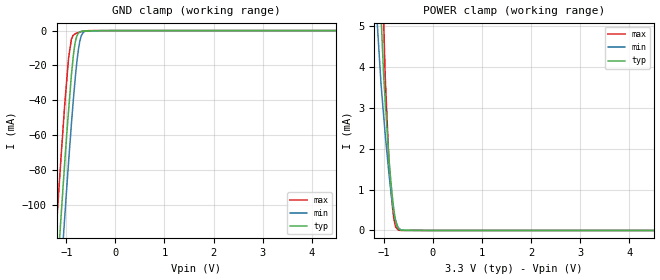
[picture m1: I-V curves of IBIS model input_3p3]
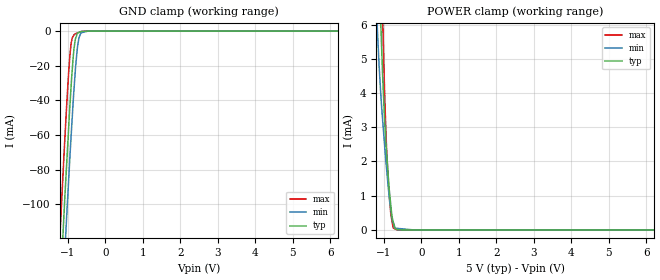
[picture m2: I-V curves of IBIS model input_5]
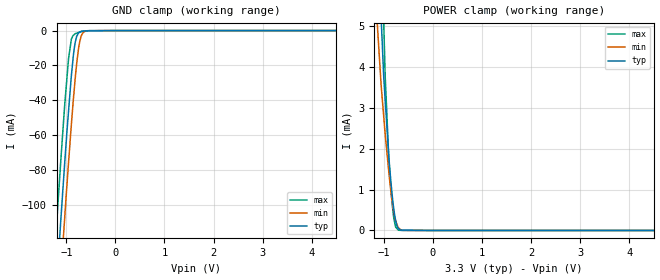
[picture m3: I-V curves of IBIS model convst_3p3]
|Texas Instruments Incorporated
| 18 Bit 1MSPS Parallel ADC W/Ref, Pseudo Bipolar, Fully Differential Input
| Marketing part#   Digital Voltage Range   Package-type   #pins
| ADS8482IBRGZR   2.7 - 5.25V   VQFN   48
| ADS8482IBRGZRG4   2.7 - 5.25V   VQFN   48
| ADS8482IBRGZT   2.7 - 5.25V   VQFN   48
| ADS8482IBRGZTG4   2.7 - 5.25V   VQFN   48
| ADS8482IRGZR   2.7 - 5.25V   VQFN   48
| ADS8482IRGZRG4   2.7 - 5.25V   VQFN   48
| ADS8482IRGZT   2.7 - 5.25V   VQFN   48
| ADS8482IRGZTG4   2.7 - 5.25V   VQFN   48
[IBIS Ver]   3.2
[File name]   ads8482.ibs
|SIMDE Ver   V2.2 - 201009 - RHL4 - Build 424
[File Rev]   1.1
[Date]   03/11/2011
[Source]
| Texas Instruments Incorporated.
| Analog-eLab Design Center, HPA
| 12500 TI Blvd
| Dallas, TX -75243
| e-mail: elab_ibis@list.ti.com
| -Model generated from simulations in TISPICE
[Notes]   Revision History:
| Rev 1.0: 1/21/2011
| - Initial version of the model
| - Model generated from simulations in TISPICE
| - Model matched to SPICE simulation
| - C_comp although listed in numerical order of value are
|   obtained from varying PVT conditions. For PVT conditions for
|   each specific value refer the buffer description under
|   respective [Model]. IBIS model user is responsible for using
|   appropriate C_comp to simulate for Signal Integrity.
| - Model names with a trailing _3p3 contains
|   the model for 3.3V [3.0V and 3.6V]. Model names with trailing _5
|   contains the model for 5.0V [4.75V and 5.25V] operation.
| Rev 1.1: 03/11/2011
| - Updated copyright to 2011
[Disclaimer]
| This model is designed as an aid for customers of Texas Instruments.
| TI and its licensors and suppliers make no warranties, either expressed
| or implied, with respect to this  model, including the warranties of
| merchantability or fitness for a particular purpose. The model is
| provided solely on an "as is" basis. The entire risk as to its quality
| and performance is with the customer.
[Copyright]
 (C) Copyright 2011 Texas Instruments Incorporated.All rights reserved.
|   ADS8482
[Component]   ADS8482
[Manufacturer]   TI
[Package]   |48 VQFN -  RGZ package
|   typ   min   max
R_pkg   0.08052   0.03771   0.10186
L_pkg   1.45674nH   0.98129nH   1.85620nH
C_pkg   0.15530pF   0.13533pF   0.18669pF
[Pin]  signal_name   model_name   R_pin   L_pin   C_pin
1   VBD   POWER   0.09317   1.68150nH  0.14766pF
2   BUS18/_16   input   0.08577   1.52984nH  0.15866pF
3   BYTE   input   0.07932   1.40125nH  0.15118pF
4   _CONVST   convst   0.03771   0.98129nH  0.18224pF
5   _RD   input   0.07064   1.23015nH  0.14114pF
6   _CS   input   0.06907   1.19953nH  0.13533pF
7   VA   POWER   0.06918   1.20163nH  0.13515pF
8   AGND   GND   0.06936   1.20524nH  0.13665pF
9   AGND   GND   0.07148   1.24671nH  0.13959pF
10   VA   POWER   0.07551   1.32594nH  0.14513pF
11   REFM   GND   0.08138   1.44284nH  0.15299pF
12   REFM   GND   0.08851   1.58840nH  0.14292pF
13   REFIN   TERM   0.04791   1.34371nH  0.18669pF
14   REFOUT   TERM   0.09373   1.68884nH  0.16643pF
15   NC   NC   0.08818   1.57624nH  0.15943pF
16   VA   POWER   0.08376   1.48731nH  0.15367pF
17   AGND   GND   0.08064   1.42465nH  0.14967pF
18   IN(+)   TERM   0.07903   1.39192nH  0.14762pF
19   IN(-)   TERM   0.07908   1.39202nH  0.14763pF
20   AGND   GND   0.08076   1.42454nH  0.14974pF
21   VA   POWER   0.08394   1.48721nH  0.15381pF
22   VA   POWER   0.08845   1.57664nH  0.15955pF
23   AGND   GND   0.09404   1.68894nH  0.16459pF
24   AGND   GND   0.09491   1.71030nH  0.14731pF
25   VA   POWER   0.04541   1.19009nH  0.19066pF
26   AGND   GND   0.08580   1.52394nH  0.16244pF
27   AGND   GND   0.04036   1.03065nH  0.19517pF
28   DB17   db   0.07628   1.33321nH  0.14727pF
29   DB16   db   0.07240   1.25624nH  0.14061pF
30   DB15   db   0.07047   1.21832nH  0.13804pF
31   DB14   db   0.07072   1.22312nH  0.13834pF
32   DB13   db   0.07310   1.27024nH  0.14147pF
33   DB12   db   0.07738   1.35501nH  0.14714pF
34   DB11   db   0.08319   1.47074nH  0.15496pF
35   DB10   db   0.09018   1.61144nH  0.16452pF
36   VBD   POWER   0.04686   1.31549nH  0.18631pF
37   BDGND   GND   0.04818   1.32883nH  0.18833pF
38   DB9   db   0.10081   1.82484nH  0.17209pF
39   DB8   db   0.09486   1.70495nH  0.16715pF
40   DB7   db   0.08995   1.60681nH  0.16090pF
41   DB6   db   0.08626   1.53385nH  0.15618pF
42   DB5   db   0.08401   1.48973nH  0.15334pF
43   DB4   db   0.08333   1.47703nH  0.15250pF
44   DB3   db   0.08427   1.49644nH  0.15371pF
45   DB2   db   0.08677   1.54701nH  0.15692pF
46   DB1   db   0.09066   1.62564nH  0.16196pF
47   DB0   db   0.09576   1.72934nH  0.16839pF
48   BUSY   busy   0.10186   1.85620nH  0.15594pF
[Pin Mapping]  pulldown_ref pullup_ref gnd_clamp_ref power_clamp_ref
1   NC   PWRBUS1
2   GNDBUS1   PWRBUS1
3   GNDBUS1   PWRBUS1
4   GNDBUS1   PWRBUS1
5   GNDBUS1   PWRBUS1
6   GNDBUS1   PWRBUS1
7   NC   PWRBUS2
8   GNDBUS2   NC
9   GNDBUS2   NC
10   NC   PWRBUS2
11   GNDBUS3   NC
12   GNDBUS3   NC
13   GNDBUS2   PWRBUS2
14   GNDBUS2   PWRBUS2
15   NC   NC
16   NC   PWRBUS2
17   GNDBUS2   NC
18   GNDBUS2   PWRBUS2
19   GNDBUS2   PWRBUS2
20   GNDBUS2   NC
21   NC   PWRBUS2
22   NC   PWRBUS2
23   GNDBUS2   NC
24   GNDBUS2   NC
25   NC   PWRBUS2
26   GNDBUS2   NC
27   GNDBUS2   NC
28   GNDBUS1   PWRBUS1
29   GNDBUS1   PWRBUS1
30   GNDBUS1   PWRBUS1
31   GNDBUS1   PWRBUS1
32   GNDBUS1   PWRBUS1
33   GNDBUS1   PWRBUS1
34   GNDBUS1   PWRBUS1
35   GNDBUS1   PWRBUS1
36   NC   PWRBUS1
37   GNDBUS1   NC
38   GNDBUS1   PWRBUS1
39   GNDBUS1   PWRBUS1
40   GNDBUS1   PWRBUS1
41   GNDBUS1   PWRBUS1
42   GNDBUS1   PWRBUS1
43   GNDBUS1   PWRBUS1
44   GNDBUS1   PWRBUS1
45   GNDBUS1   PWRBUS1
46   GNDBUS1   PWRBUS1
47   GNDBUS1   PWRBUS1
48   GNDBUS1   PWRBUS1
|   Model Selectors
[Model Selector] input
input_3p3   3.3V digital input
input_5   5.0V digital input
[Model Selector] convst
convst_3p3   3.3V digital input
convst_5   5.0V digital input
[Model Selector] busy
busy_3p3   3.3V digital output
busy_5   5.0V digital output
[Model Selector] db
db_3p3   3.3V 3-state output
db_5   5.0V 3-state output
[Model Selector] TERM
TERM_3p3  3.3V nominal termination
TERM_5   5.0V nominal termination
[Model]  TERM_3p3
Model_type Terminator
C_comp   1.0e-20F  1.0e-20F  1.0e-20F
|   typ   min   max
[Voltage Range]   3.3V   3.0V   3.6V
[POWER Clamp Reference]   3.3V   3.0V   3.6V
[GND Clamp Reference]   0V   0V   0V
|Ambient Temperature   25   85   -40
|Junction Temperature
[Temperature Range]   30   90   -40
[Model]  TERM_5
Model_type Terminator
C_comp   1.0e-20F  1.0e-20F  1.0e-20F
|   typ   min   max
[Voltage Range]   5.0V   4.75V   5.25V
[POWER Clamp Reference]   5.0V   4.75V   5.25V
[GND Clamp Reference]   0V   0V   0V
|Ambient Temperature   25   85   -40
|Junction Temperature
[Temperature Range]   30   90   -40
| Models and submodels in the file (10): input_3p3 (Input), input_5 (Input), convst_3p3 (Input), convst_5 (Input), busy_3p3 (Output), busy_5 (Output), db_3p3 (3-state), db_5 (3-state), TERM_3p3 (Terminator), TERM_5 (Terminator)
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|   input_3p3 Model
[Model]   input_3p3
Model_type   Input
Vinl = 0.8
Vinh = 2.3
|   typ   min   max
|   (nom PVT)   (Fast PVT)   (slow PVT)
|C_comp from frequency method(F=1MHz)
|Average
|C_comp   1.211e-12   1.085e-12   1.349e-12
|C_comp from L-C Tank method(L=1nH)
|Resonant Frequency(Hz)   5.36e9   5.44e9   5.26e9
C_comp   8.826e-13   8.568e-13   9.164e-13
| Where nom  PVT is Nominal Process,  3.3V,  30C
|   Fast PVT is Strong Process,   3.6V,  -40C
|   Slow PVT is Weak Process,   3V,  90C
[Model Spec]
Vinl   0.8   0.8   0.8
Vinh   2.3   2.0   2.6
[Voltage Range]   3.3   3   3.6
|Ambient Temperature   25   85   -40
|Junction Temperature
[Temperature Range]   30   90   -40
[Power Clamp Reference]   3.3   3   3.6
[GND Clamp Reference]   0   0   0
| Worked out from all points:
|   GND clamp passes 1 mA (typ) near -0.73 V on its own axis
|   POWER clamp passes 1 mA (typ) near -0.84 V on its own axis
[GND Clamp]
|   Voltage   I(typ)   I(min)   I(max)
-3.3V     -1.107A    -1.129A    -1.081A
-1.287V   -183.7mA   -214.7mA   -150.2mA
-1.159V   -128.6mA   -159.6mA   -94.06mA
-1.137V   -119mA     -150.1mA   -84.7mA
-1.112V   -108.3mA   -139.8mA   -74.2mA
-1.033V   -75.79mA   -107.1mA   -42.53mA
-954mV    -45.81mA   -75.15mA   -15.73mA
-896.4mV  -25.43mA   -53.39mA   -4.841mA
-810mV    -5.66mA    -24.62mA   -1.68mA
-723mV    -836.2uA   -5.772mA   -858.6uA
-591mV    -229.6uA   -174.9uA   -164.1uA
6.6V      0A         0A         0A
[POWER Clamp]
|   Voltage   I(typ)   I(min)   I(max)
-3.3V     114.3mA    94.22mA    142.1mA
-1.158V   9.058mA    5.513mA    13.01mA
-1.096V   6.558mA    4.315mA    9.552mA
-1.055V   5.194mA    3.537mA    7.319mA
-1.003V   3.763mA    2.793mA    5.098mA
-972mV    3.176mA    2.343mA    3.755mA
-896.4mV  1.759mA    1.395mA    1.692mA
-874.8mV  1.454mA    1.156mA    1.298mA
-795.6mV  513.3uA    430.3uA    288.7uA
-745.8mV  160.8uA    193uA      65.47uA
-702mV    45.96uA    64.11uA    6.738uA
6.6V      0A         0A         0A
|   input_5 Model
[Model]   input_5
Model_type   Input
Vinl = 0.8
Vinh = 4.0
|   typ   min   max
|   (nom PVT)   (Fast PVT)   (slow PVT)
|C_comp from frequency method(F=1MHz)
|Average
|C_comp   1.113e-12   1.007e-12   1.226e-12
|C_comp from L-C Tank method(L=1nH)
|Resonant Frequency(Hz)   5.52e9   5.6e9   5.42e9
C_comp   8.321e-13   8.085e-13   8.631e-13
| Where nom  PVT is Nominal Process,  5V,  30C
|   Fast PVT is Strong Process,   5.25V,  -40C
|   Slow PVT is Weak Process,   4.75V,  90C
[Model Spec]
Vinl   0.8   0.8   0.8
Vinh   4.0   3.75   4.25
[Voltage Range]   5   4.75   5.25
|Ambient Temperature   25   85   -40
|Junction Temperature
[Temperature Range]   30   90   -40
[Power Clamp Reference]   5   4.75   5.25
[GND Clamp Reference]   0   0   0
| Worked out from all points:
|   GND clamp passes 1 mA (typ) near -0.73 V on its own axis
|   POWER clamp passes 1 mA (typ) near -0.84 V on its own axis
[GND Clamp]
|   Voltage   I(typ)   I(min)   I(max)
-5V       -1.898A    -1.916A    -1.876A
-1.306V   -192.2mA   -223.1mA   -158.4mA
-1.108V   -106.7mA   -138mA     -72.38mA
-1.08V    -94.88mA   -126.2mA   -61.18mA
-1.04V    -78.88mA   -109.4mA   -44.94mA
-950.3mV  -43.75mA   -73.69mA   -14.72mA
-913.5mV  -31.06mA   -60mA      -6.967mA
-840mV    -10.48mA   -34.09mA   -2.163mA
-745.8mV  -1.183mA   -9.257mA   -1.102mA
-707.7mV  -789.6uA   -4.052mA   -791.6uA
-640mV    -158.4uA   -951.7uA   -242uA
10V       0A         0A         0A
[POWER Clamp]
|   Voltage   I(typ)   I(min)   I(max)
-5V       200.2mA    168.8mA    246.3mA
-1.178V   10.06mA    6.005mA    13.91mA
-1.08V    6.013mA    3.952mA    8.603mA
-1.064V   5.51mA     3.682mA    7.807mA
-1.035V   4.599mA    3.255mA    6.396mA
-990mV    3.456mA    2.619mA    4.468mA
-929.3mV  2.319mA    1.811mA    2.435mA
-876.8mV  1.492mA    1.196mA    1.331mA
-813.7mV  723.3uA    596.6uA    459.2uA
-750.8mV  240uA      226.2uA    58.49uA
-640.5mV  4.904uA    46.48uA    457nA
10V       0A         0A         0A
|   convst_3p3 Model
[Model]   convst_3p3
Model_type   Input
Vinl = 0.8
Vinh = 2.3
|   typ   min   max
|   (nom PVT)   (Fast PVT)   (slow PVT)
|C_comp from frequency method(F=1MHz)
|Average
|C_comp   1.462e-12   1.335e-12   1.599e-12
|C_comp from L-C Tank method(L=1nH)
|Resonant Frequency(Hz)   4.68e9   4.75e9   4.61e9
C_comp   1.158e-12   1.124e-12   1.193e-12
| Where nom  PVT is Nominal Process,  3.3V,  30C
|   Fast PVT is Strong Process,   3.6V,  -40C
|   Slow PVT is Weak Process,   3V,  90C
[Model Spec]
Vinl   0.8   0.8   0.8
Vinh   2.3   2.0   2.6
[Voltage Range]   3.3   3   3.6
|Ambient Temperature   25   85   -40
|Junction Temperature
[Temperature Range]   30   90   -40
[Power Clamp Reference]   3.3   3   3.6
[GND Clamp Reference]   0   0   0
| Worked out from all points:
|   GND clamp passes 1 mA (typ) near -0.73 V on its own axis
|   POWER clamp passes 1 mA (typ) near -0.84 V on its own axis
[GND Clamp]
|   Voltage   I(typ)   I(min)   I(max)
-3.3V     -1.107A    -1.129A    -1.081A
-1.287V   -183.7mA   -214.7mA   -150.2mA
-1.159V   -128.6mA   -159.6mA   -94.06mA
-1.137V   -119mA     -150.1mA   -84.7mA
-1.112V   -108.3mA   -139.8mA   -74.2mA
-1.033V   -75.79mA   -107.1mA   -42.53mA
-954mV    -45.81mA   -75.15mA   -15.73mA
-896.4mV  -25.43mA   -53.39mA   -4.841mA
-810mV    -5.66mA    -24.62mA   -1.68mA
-723mV    -836.2uA   -5.772mA   -858.6uA
-591mV    -229.6uA   -174.9uA   -164.1uA
6.6V      0A         0A         0A
[POWER Clamp]
|   Voltage   I(typ)   I(min)   I(max)
-3.3V     114.3mA    94.22mA    142.1mA
-1.158V   9.058mA    5.513mA    13.01mA
-1.096V   6.558mA    4.315mA    9.552mA
-1.055V   5.194mA    3.537mA    7.319mA
-1.003V   3.763mA    2.793mA    5.098mA
-972mV    3.176mA    2.343mA    3.755mA
-896.4mV  1.759mA    1.395mA    1.692mA
-874.8mV  1.454mA    1.156mA    1.298mA
-795.6mV  513.3uA    430.3uA    288.7uA
-745.8mV  160.8uA    193uA      65.47uA
-702mV    45.96uA    64.11uA    6.738uA
6.6V      0A         0A         0A
